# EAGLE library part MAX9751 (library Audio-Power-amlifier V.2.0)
The MAX9751 combine a stereo, 2.6W audio power amplifier and stereo DirectDrive® 110mW headphone amplifier in a single device. The headphone amplifier uses Maxim’s DirectDrive architecture that produces a ground-referenced output from a single supply, eliminating the need for large DC-blocking capacitors, saving cost, space, and component height. A high 90dB PSRR and low 0.01% THD+N ensures clean, low-distortion amplification of the audio signal.
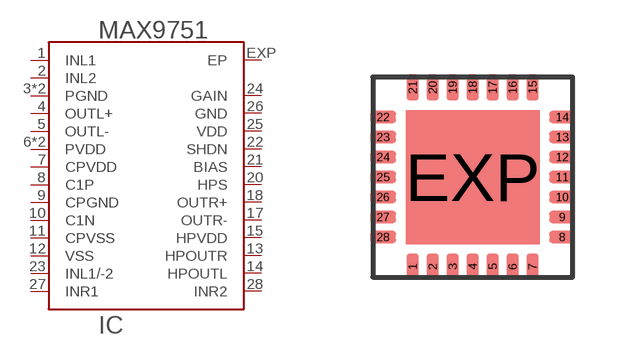
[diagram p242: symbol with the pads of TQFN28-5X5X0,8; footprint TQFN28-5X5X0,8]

Designator prefix IC

## MAX9751  [TQFN28-5X5X0,8]
1  INL1  in
2  INL2  in
3  PGND  pwr
4  OUTL+  out
5  OUTL-  out
6  PVDD  pwr
7  CPVDD  pwr
8  C1P
9  CPGND  pwr
10  C1N  in
11  CPVSS  pwr
12  VSS  pwr
13  HPOUTR  out
14  HPOUTL  out
15  HPVDD  pwr
16  PVDD  pwr
17  OUTR-  out
18  OUTR+  out
19  PGND  pwr
20  HPS  in
21  BIAS
22  SHDN
23  INL1/-2  in
24  GAIN  in
25  VDD  pwr
26  GND  pwr
27  INR1  in
28  INR2  in
EXP  EP  pwr

## Footprint TQFN28-5X5X0,8 (pad centres in mm)
TQFN28-5x5x0,8 Source: www.maxim-ic.com/packages
smd 0.305 x 0.65: 1 -1.5,-2.24; 2 -1,-2.24; 3 -0.5,-2.24; 4 0,-2.24; 5 0.5,-2.24; 6 1,-2.24; 7 1.5,-2.24; 15 1.5,2.24; 16 1,2.24; 17 0.5,2.24; 18 0,2.24; 19 -0.5,2.24; 20 -1,2.24; 21 -1.5,2.24
smd 0.65 x 0.305: 8 2.24,-1.5; 9 2.24,-1; 10 2.24,-0.5; 11 2.24,0; 12 2.24,0.5; 13 2.24,1; 14 2.24,1.5; 22 -2.24,1.5; 23 -2.24,1; 24 -2.24,0.5; 25 -2.24,0; 26 -2.24,-0.5; 27 -2.24,-1; 28 -2.24,-1.5
smd 3.35 x 3.35: EXP 0,0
